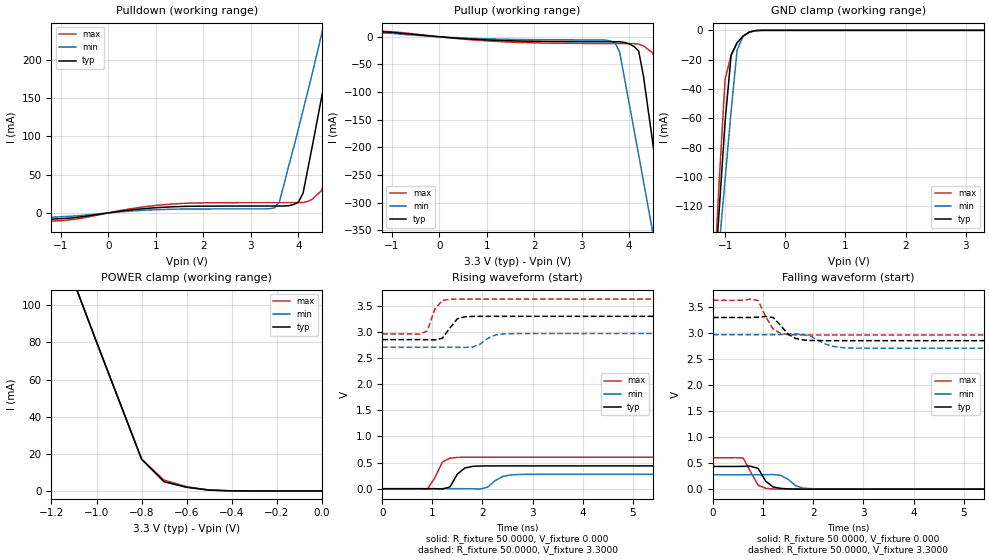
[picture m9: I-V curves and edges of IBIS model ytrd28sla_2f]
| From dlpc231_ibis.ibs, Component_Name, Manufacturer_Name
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| Model ytrd28sla_2f
[Model]   ytrd28sla_2f
Model_type   3-state
Polarity   Non-Inverting
Enable   Active-High
Vmeas = 1.5000V
Cref =50.0000pF
Rref = 0.5000k
Vref =  0.000V
C_comp   0.7000pF   0.7000pF   0.7000pF
[Temperature Range]   25.0000   0.1240k   -40.0000
[Voltage Range]   3.3000V   2.9700V   3.6300V
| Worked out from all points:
|   slope of the pulldown table from 0 to 0.495 V, typ, clamps not added: 125 ohm
|   slope of the pullup table from 0 to 0.495 V, typ, clamps not added: 154 ohm
|   GND clamp passes 1 mA (typ) near -0.57 V on its own axis
|   POWER clamp passes 1 mA (typ) near -0.54 V on its own axis
|   rising waveform, R_fixture 50.0000, V_fixture 0.000: 20-80 % time 205ps typ, 247ps min, 197ps max; typ from 0 V to 0.437 V
|   rising waveform, R_fixture 50.0000, V_fixture 3.3000: 20-80 % time 215ps typ, 262ps min, 175ps max; typ from 2.85 V to 3.3 V
|   falling waveform, R_fixture 50.0000, V_fixture 0.000: 20-80 % time 208ps typ, 245ps min, 208ps max; typ from 0.437 V to 0 V
|   falling waveform, R_fixture 50.0000, V_fixture 3.3000: 20-80 % time 276ps typ, 348ps min, 225ps max; typ from 3.3 V to 2.85 V
[Pulldown]
-3.3V     -12mA      -10mA      -15mA
1.4V      8.055mA    4.828mA    11.75mA
3.5V      8.95mA     6.53mA     13.38mA
3.6V      8.957mA    14.27mA    13.39mA
4V        13.9mA     108.9mA    13.43mA
4.1V      25.78mA    133.4mA    13.62mA
4.2V      57.42mA    158.3mA    14.96mA
4.5V      154mA      235.7mA    29.88mA
4.7V      221.2mA    290.1mA    107mA
4.9V      290.8mA    347.4mA    190.8mA
5.1V      363.2mA    408.4mA    277.3mA
6.6V      1.036A     959.4mA    1.038A
[Pullup]
-3.3V     7mA        9.3mA      5mA
-1.7V     11.3mA     9.5mA      11.8mA
1.3V      -6.71mA    -4.429mA   -8.856mA
3.7V      -8.961mA   -10.76mA   -12.3mA
3.8V      -9.174mA   -27.88mA   -12.33mA
4.2V      -25.8mA    -214mA     -13.32mA
4.3V      -70.86mA   -260.9mA   -16.36mA
4.5V      -194mA     -355.2mA   -29.61mA
4.7V      -318.2mA   -450.2mA   -92.76mA
4.9V      -443.3mA   -545.8mA   -248.8mA
5.1V      -569mA     -641.8mA   -405.8mA
6.6V      -1.524A    -1.372A    -1.596A
[GND_clamp]
-3.3V     -1.515A    -1.204A    -1.847A
-1.2V     -185.5mA   -194.5mA   -182.5mA
-1.1V     -123.8mA   -147.9mA   -104.5mA
-1V       -62.37mA   -101.6mA   -33.38mA
-900mV    -16.91mA   -55.06mA   -16.91mA
-800mV    -8.434mA   -13.38mA   -8.434mA
-700mV    -3.946mA   -3.946mA   -3.946mA
-600mV    -1.264mA   -1.264mA   -1.264mA
-500mV    -213uA     -246.3uA   -196.1uA
-400mV    -14.84uA   -26.5uA    -10.46uA
3.3V      3.366nA    3.366nA    16.84nA
[POWER_clamp]
-3.3V     1.025A     838.2mA    1.218A
-1.1V     112.5mA    112.5mA    112.5mA
-1V       80.27mA    80.27mA    80.27mA
-800mV    17.07mA    17.07mA    17.07mA
-700mV    4.946mA    4.946mA    5.793mA
-600mV    1.98mA     1.98mA     2.27mA
-500mV    443.7uA    443.7uA    443.7uA
-400mV    34.77uA    34.77uA    34.77uA
0V        3.366nA    3.366nA    56.62nA
[Ramp]
dV/dt_r   0.2620/0.1821n   0.1658/0.2348n   0.3620/0.1546n
dV/dt_f   0.2676/0.2488n   0.1566/0.3276n   0.4002/0.2097n
R_load = 50.0000
[Rising Waveform]
R_fixture = 50.0000
V_fixture = 0.000
V_fixture_min = 0.000
V_fixture_max = 0.000
0s        0V         0V         0V
900ps     146.1uV    -1.246uV   -8.761mV
1.2ns     -4.897mV   -1.784uV   511.1mV
1.35ns    33.31mV    44.49uV    584.2mV
1.5ns     282.4mV    228.3uV    599.6mV
1.65ns    396.9mV    259.5uV    602.8mV
1.95ns    434.4mV    -7.017mV   603.4mV
2.4ns     436.7mV    232.4mV    603.4mV
2.7ns     436.7mV    271.9mV    603.4mV
14.85ns   436.7mV    276.4mV    603.4mV
[Rising Waveform]
R_fixture = 50.0000
V_fixture = 3.3000
V_fixture_min = 2.9700
V_fixture_max = 3.6300
0s        2.854V     2.709V     2.963V
900ps     2.853V     2.709V     3.021V
1.05ns    2.848V     2.709V     3.44V
1.2ns     2.88V      2.709V     3.604V
1.35ns    3.078V     2.708V     3.626V
1.5ns     3.254V     2.707V     3.629V
1.65ns    3.291V     2.703V     3.629V
2.25ns    3.3V       2.941V     3.63V
2.55ns    3.3V       2.967V     3.63V
14.85ns   3.3V       2.97V      3.63V
[Falling Waveform]
R_fixture = 50.0000
V_fixture = 0.000
V_fixture_min = 0.000
V_fixture_max = 0.000
0s        436.7mV    276.4mV    603.4mV
600ps     438.2mV    276.3mV    597.7mV
900ps     398mV      276.9mV    73.88mV
1.05ns    153mV      278.8mV    17.33mV
1.2ns     41.26mV    280.3mV    3.836mV
1.35ns    14.97mV    266.7mV    743uV
1.65ns    1.522mV    64.41mV    29.58uV
1.8ns     432.9uV    19.49mV    6.786uV
2.25ns    9.181uV    3.708mV    0V
14.85ns   0V         0V         0V
[Falling Waveform]
R_fixture = 50.0000
V_fixture = 3.3000
V_fixture_min = 2.9700
V_fixture_max = 3.6300
0s        3.3V       2.97V      3.63V
750ps     3.3V       2.97V      3.654V
900ps     3.306V     2.969V     3.623V
1.05ns    3.319V     2.969V     3.314V
1.2ns     3.298V     2.97V      3.075V
1.5ns     2.975V     2.979V     2.971V
1.8ns     2.868V     2.975V     2.963V
2.4ns     2.854V     2.744V     2.963V
2.85ns    2.854V     2.711V     2.963V
14.85ns   2.854V     2.709V     2.963V
